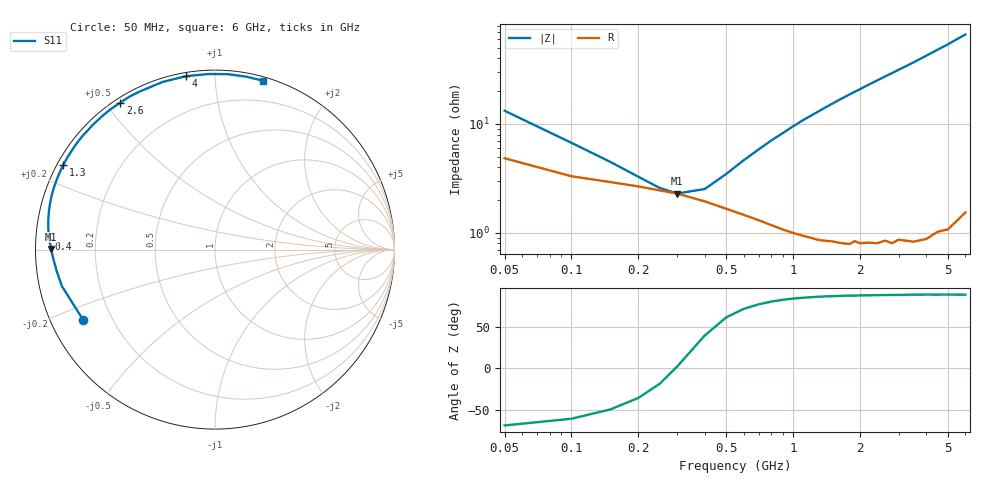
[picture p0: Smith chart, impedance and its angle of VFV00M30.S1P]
! Infineon Technologies  Discrete & RF Semiconductors
! BBY 58-03
! Si Tuning Diode in SOD323
! VR =
! S-Parameters:  June  1999
# GHz  S  MA  R  50
!  f  S11
! GHz  MAG  ANG
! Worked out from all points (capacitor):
!   34 points, 50 MHz to 6 GHz, reference 50 ohm
!   read as one part to ground: C = 241 pF near 50 MHz
!   lowest |Z| = 2.3 ohm at 300 MHz (marker M1)
!   series resonance near 295.2 MHz, so ESL is about 1.2 nH
!   S11 on the Smith chart (normalised r, x): 50 MHz: 0.10, -0.25; 400 MHz: 0.04, +0.03; 1.3 GHz: 0.02, +0.26; 2.6 GHz: 0.02, +0.55; 4 GHz: 0.02, +0.85; 6 GHz: 0.03, +1.33
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0.05  0.8326 -152.1
0.1  0.8772 -166.6
0.15  0.8898 -172.2
0.2  0.8986 -175.6
0.25  0.9064 -178.1
0.3  0.9121 179.8
0.4  0.9251 176.3
0.5  0.9357 173.0
0.6  0.9435 169.9
0.8  0.9548 164.1
0.9  0.959 161.4
1.1  0.9645 155.9
1.3  0.9682 150.9
1.4  0.9691 148.4
1.6  0.971 143.6
1.8  0.9726 139.1
2  0.9729 134.8
2.2  0.9735 130.6
2.4  0.9746 126.7
2.6  0.9741 122.8
2.8  0.9763 119.2
3  0.9755 115.6
3.5  0.9786 107.4
4  0.9797 99.4
4.5  0.9789 92.2
5  0.9802 85.8
5.5  0.979 79.5
6  0.9779 74.0
